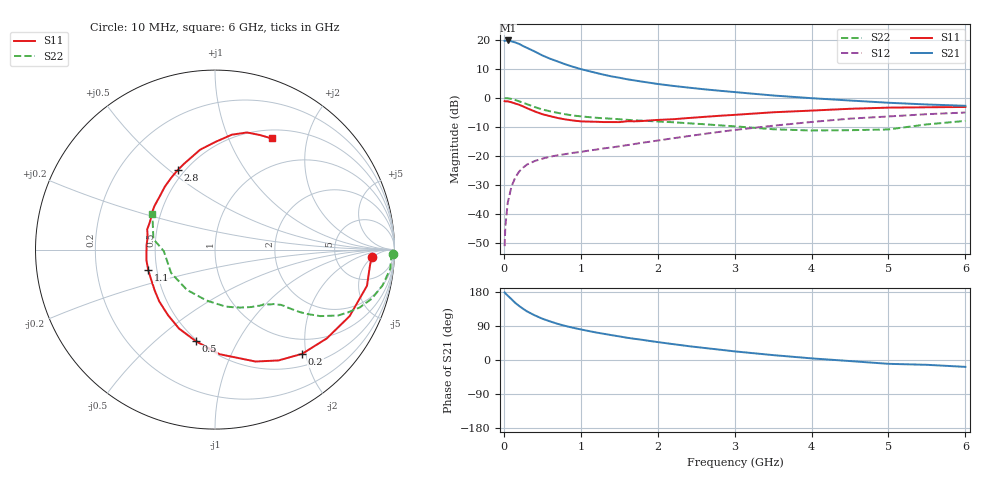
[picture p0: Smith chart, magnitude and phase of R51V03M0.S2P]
! SIEMENS Small Signal Semiconductors
! BFR183
! Si NPN RF Bipolar Junction Transistor in SOT23
! VCE = 1 V  IC = 3 mA
! Common Emitter S-Parameters:  May  1996
# GHz  S  MA  R  50
!  f  S11  S21  S12  S22
! GHz  MAG  ANG  MAG  ANG  MAG  ANG  MAG  ANG
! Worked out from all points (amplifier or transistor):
!   36 points, 10 MHz to 6 GHz, reference 50 ohm
!   highest |S21| = 19.7 dB at 50 MHz (marker M1)
!   |S21| within 3 dB of that: start of sweep to 337.1 MHz
!   unconditionally stable (mu >= 1): 1.201 GHz to 2.959 GHz
!   at 250 MHz: K = 0.30, MSG = 20.9 dB, |S12| = -24.1 dB
!   at 1.4 GHz: K = 1.06, MAG = 10.7 dB, |S12| = -17.1 dB
!   at 6 GHz: K = 0.94, MSG = 1.2 dB, |S12| = -5.1 dB
!   S11 on the Smith chart (normalised r, x): 10 MHz: 14, -5; 200 MHz: 0.71, -1.93; 500 MHz: 0.49, -0.69; 1.1 GHz: 0.45, -0.12; 2.8 GHz: 0.46, +0.54; 6 GHz: 0.61, +1.45
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0.01  0.8758 -2.6  9.549 178.3  0.0028 90.1  0.9929 -1.3
0.02  0.8682 -5.5  9.596 175.9  0.0062 90.2  0.9829 -2.4
0.05  0.8705 -13.4  9.685 170.0  0.0155 82.4  0.9823 -6.3
0.1  0.8367 -26.3  9.327 160.4  0.03 76.1  0.9543 -12.1
0.15  0.7953 -38.5  8.934 150.5  0.0428 69.8  0.915 -17.4
0.2  0.7569 -50.1  8.427 142.4  0.054 64.7  0.8683 -21.8
0.25  0.7117 -60.2  7.771 135.2  0.0627 59.8  0.8205 -25.2
0.3  0.6632 -70.1  7.232 128.4  0.0709 56.7  0.7774 -28.2
0.4  0.5837 -87.4  6.264 118.0  0.0816 51.3  0.6935 -32.3
0.5  0.522 -101.6  5.355 109.0  0.0896 48.1  0.6292 -34.8
0.6  0.4835 -114.5  4.707 101.9  0.0969 46.3  0.586 -36.4
0.7  0.449 -125.8  4.211 95.4  0.1024 45.4  0.5504 -37.5
0.8  0.4241 -137.1  3.763 89.9  0.1074 44.9  0.52 -38.5
1.1  0.3891 -162.9  2.888 76.6  0.1233 46.4  0.4653 -41.2
1.3  0.382 -177.8  2.491 69.1  0.1347 47.1  0.4438 -43.1
1.6  0.3941 163.4  2.085 58.8  0.153 48.9  0.418 -47.0
2.2  0.4276 136.0  1.601 41.9  0.201 50.2  0.3793 -57.5
2.8  0.4895 115.1  1.323 27.4  0.2587 47.8  0.3358 -72.8
3.5  0.563 98.4  1.095 12.9  0.3303 41.1  0.2876 -99.5
4.5  0.6468 81.7  0.897 -2.8  0.4377 28.9  0.2769 -152.0
5.5  0.6862 68.3  0.767 -12.7  0.5219 15.9  0.3485 170.2
6  0.6948 63.0  0.728 -18.1  0.5579 7.5  0.4001 150.6
